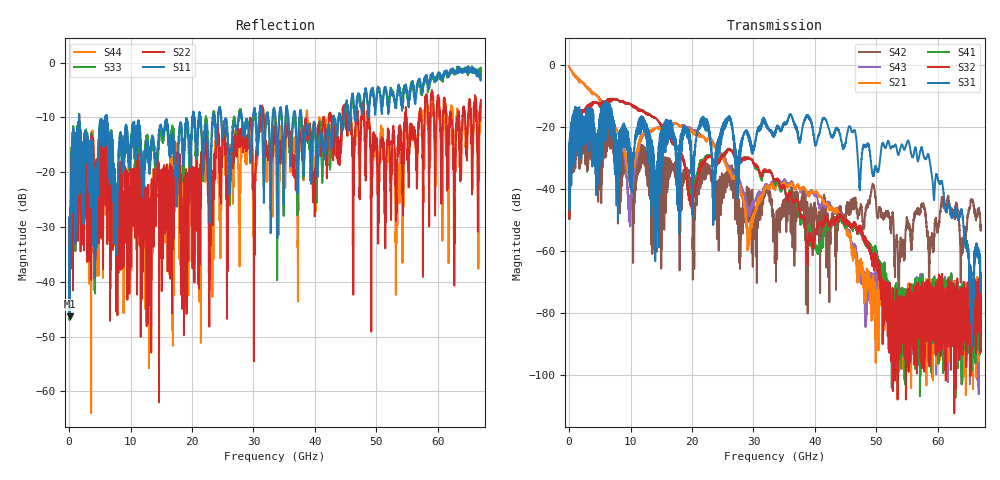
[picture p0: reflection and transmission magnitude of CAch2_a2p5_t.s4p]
!Agilent Technologies,N5247A,US51170199,A.09.90.13
!Agilent N5247A: A.09.90.13
!Date: Tuesday, October 23, 2018 14:23:46
!Correction: S11(Full 4 Port(1,2,3,4))
!S12(Full 4 Port(1,2,3,4))
!S13(Full 4 Port(1,2,3,4))
!S14(Full 4 Port(1,2,3,4))
!S21(Full 4 Port(1,2,3,4))
!S22(Full 4 Port(1,2,3,4))
!S23(Full 4 Port(1,2,3,4))
!S24(Full 4 Port(1,2,3,4))
!S31(Full 4 Port(1,2,3,4))
!S32(Full 4 Port(1,2,3,4))
!S33(Full 4 Port(1,2,3,4))
!S34(Full 4 Port(1,2,3,4))
!S41(Full 4 Port(1,2,3,4))
!S42(Full 4 Port(1,2,3,4))
!S43(Full 4 Port(1,2,3,4))
!S44(Full 4 Port(1,2,3,4))
!S4P File: Measurements: <S11,S12,S13,S14>,
!<S21,S22,S23,S24>,
!<S31,S32,S33,S34>,
!<S41,S42,S43,S44>:
# Hz S  dB  R 50
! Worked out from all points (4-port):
!   6701 points, 10 MHz to 67 GHz, reference 50 ohm
!   strongest paths, dB at 10 MHz, 16.76 GHz, 33.51 GHz, 50.25 GHz, 67 GHz:
!     S31: -33.3, -23.1, -21.4, -34.4, -73.5
!     S32: -48.5, -24.8, -37.4, -65.6, -74.8
!     S41: -48.4, -24.7, -38.1, -61.8, -78.0
!     S21: -0.3, -18.7, -39.7, -73.1, -72.6
!     S43: -0.3, -18.9, -38.9, -75.3, -81.4
!     S42: -33.5, -32.8, -57.3, -49.0, -52.8
!   lowest |S11| = -46.3 dB at 89.99 MHz (marker M1), VSWR 1.01, Z = 50.3 - j0.4 ohm
!   |S11| at or under -10 dB: 1.643 GHz to 5.891 GHz (4.247 GHz wide, 113 % of centre); 6.101 GHz to 20.05 GHz (13.95 GHz wide, 107 % of centre); 37.85 GHz to 43.09 GHz (5.244 GHz wide, 13 % of centre)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
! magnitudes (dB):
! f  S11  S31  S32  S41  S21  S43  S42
! 10 MHz  -28.4  -33.3  -48.5  -48.4  -0.3  -0.3  -33.5
! 89.99 MHz  -46.3  -33.2  -43.3  -43.2  -0.8  -0.8  -33.5
! 7.749 GHz  -35.1  -34.8  -11.0  -11.1  -21.0  -20.9  -36.7
! 9.849 GHz  -17.2  -37.6  -12.5  -12.5  -36.2  -47.8  -33.5
! 19.59 GHz  -15.3  -23.4  -43.3  -41.4  -20.7  -20.1  -36.6
! 55.13 GHz  -6.9  -24.3  -85.8  -78.5  -88.0  -70.8  -51.6
! 67 GHz  -2.1  -73.5  -74.8  -78.0  -72.6  -81.4  -52.8
